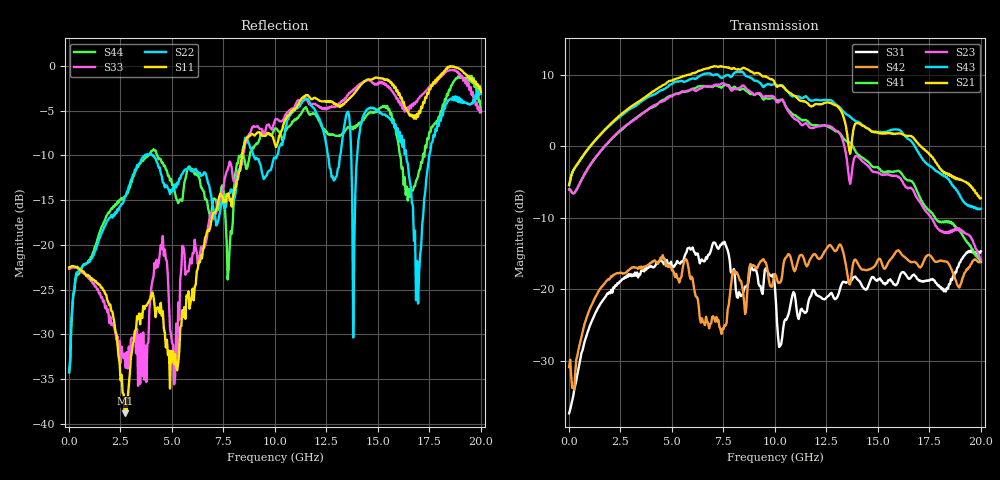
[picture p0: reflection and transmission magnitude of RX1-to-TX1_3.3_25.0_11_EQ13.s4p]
!Agilent Technologies,N5225A,MY51451112,A.09.50.13
!Agilent N5225A: A.09.50.13
!Date: Wednesday, January 31, 2018 11:05:45
!Correction: S11(Full 4 Port(1,2,3,4))
!S12(Full 4 Port(1,2,3,4))
!S13(Full 4 Port(1,2,3,4))
!S14(Full 4 Port(1,2,3,4))
!S21(Full 4 Port(1,2,3,4))
!S22(Full 4 Port(1,2,3,4))
!S23(Full 4 Port(1,2,3,4))
!S24(Full 4 Port(1,2,3,4))
!S31(Full 4 Port(1,2,3,4))
!S32(Full 4 Port(1,2,3,4))
!S33(Full 4 Port(1,2,3,4))
!S34(Full 4 Port(1,2,3,4))
!S41(Full 4 Port(1,2,3,4))
!S42(Full 4 Port(1,2,3,4))
!S43(Full 4 Port(1,2,3,4))
!S44(Full 4 Port(1,2,3,4))
!S4P File: Measurements: <S11,S12,S13,S14>,
!<S21,S22,S23,S24>,
!<S31,S32,S33,S34>,
!<S41,S42,S43,S44>:
# Hz S  RI  R 50
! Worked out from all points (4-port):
!   401 points, 10 MHz to 20 GHz, reference 50 ohm
!   strongest paths, dB at 10 MHz, 5.008 GHz, 10.01 GHz, 15 GHz, 20 GHz:
!     S21: -5.4, 9.2, 8.8, 1.9, -7.3
!     S43: -5.5, 8.7, 8.7, 2.0, -8.7
!     S23: -6.1, 7.0, 6.7, -3.7, -15.9
!     S41: -6.1, 7.1, 6.6, -2.9, -16.1
!     S42: -30.9, -17.4, -17.8, -15.9, -16.2
!     S31: -37.3, -17.1, -19.8, -18.6, -14.7
!   lowest |S11| = -38.8 dB at 2.709 GHz (marker M1), VSWR 1.02, Z = 49.1 - j0.72 ohm
!   |S11| at or under -10 dB: start of sweep to 8.414 GHz
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1e7  -0.0747 -0.00282  3.16e-05 0.000529  0.0141 0.000537  -0.000414 0.000395
     0.5361 0.0136  -0.0137 0.0139  -0.498 -0.00219  0.0263 0.0119
     0.0136 0.000859  -0.000206 0.000357  -0.0733 -0.00429  -3.11e-06 0.000307
     -0.498 -0.00171  0.0259 0.0123  0.5334 0.0128  -0.0127 0.0146
2.70865e9  -0.00877 -0.00733  0.0158 0.0034  0.0517 0.11  0.0175 0.00071
           1.457 -0.9705  0.1827 0.0164  -1.103 0.82  0.1004 0.092
           0.0582 0.107  0.019 0.00396  0.00604 0.0239  0.021 0.000704
           -0.9717 0.9521  0.0882 0.0948  1.19 -1.226  0.1832 -0.0339
6.956525e9  -0.0341 0.1407  0.0135 -0.0155  0.1409 0.0606  0.0107 -0.0273
            -3.568 0.3311  0.104 -0.1339  2.548 -0.6322  0.0258 0.0307
            0.1517 0.1341  0.0205 -0.014  0.0262 0.145  0.0239 -0.0307
            2.037 -1.591  0.0637 -0.00763  -2.594 1.785  0.0898 -0.1387
8.6057e9  0.00124 0.3855  7.93e-05 -0.00923  0.0641 0.0443  -0.00606 -0.0185
          -0.737 3.389  -0.1176 0.3736  0.0943 -2.527  -0.0111 0.1272
          0.0919 0.0504  0.00911 -0.0172  0.0264 0.3791  -0.00982 -0.0341
          -1.022 -2.214  -0.0202 0.0701  1.026 2.908  0.2071 0.1667
1.045478e10  0.1384 0.4616  -0.0275 -0.0406  0.00259 0.00713  -0.0543 -0.0121
             2.243 1.249  0.2713 0.2906  -1.943 -0.5092  0.0334 0.1828
             -0.0427 0.0417  -0.0352 -0.0383  0.2234 0.4608  -0.0595 -0.0174
             -1.92 0.5612  0.0736 0.1415  2.554 -0.2414  0.3948 -0.1052
1.415292e10  0.6636 0.4114  -0.0283 -0.00297  0.0104 0.0972  -0.0126 0.0129
             0.2482 -1.403  0.4376 0.1458  0.1227 0.8034  0.1535 0.041
             0.0223 0.1092  -0.0141 -0.00115  0.7544 0.2535  -0.0221 0.0147
             0.7433 0.411  0.1284 0.0583  -1.178 -0.8329  -0.1361 -0.4663
2e10  0.7121 0.0719  0.023 0.0347  -0.08 0.1582  0.035 0.0209
      0.055 0.4296  0.6932 0.0745  -0.0258 -0.1587  0.1546 0.0393
      -0.0784 0.1669  0.00634 0.0478  0.5637 -0.0236  0.0476 0.0206
      -0.1551 -0.0257  0.1484 0.0458  0.3558 0.0877  -0.1515 -0.5312
